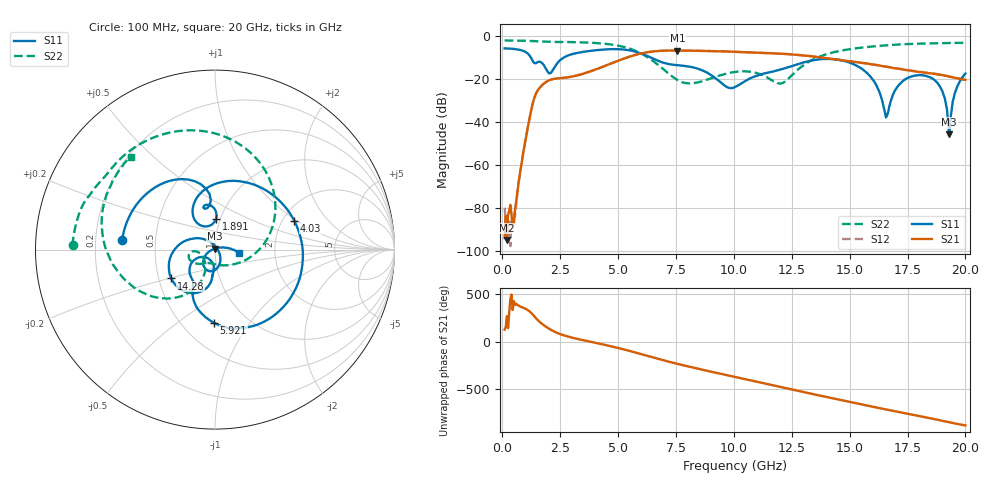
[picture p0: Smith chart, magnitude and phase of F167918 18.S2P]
!  2-Port S-parameters saved by WinCal
! VAR MeasName=S-Parameters (CALIBRATED_DATA) read from VNA (N5242A)
! VAR MeasDate=2016-11-22 10:25:39
! VAR NAME=F167918 18
! VAR FILENAME=F167918 18.S2P
! VAR DATE=2016-11-22 10:25:39
! VAR PHYS_PORTS=1,2
# Hz S DB R 50
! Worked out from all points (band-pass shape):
!   401 points, 100 MHz to 20 GHz, reference 50 ohm
!   highest |S21| = -6.67 dB at 7.562 GHz (marker M1); lowest = -94.7 dB at 199.5 MHz (marker M2)
!   |S21| within 3 dB of the highest: 5.456 GHz to 13.57 GHz (8.112 GHz wide, 85.3 % of centre)
!   lowest |S11| = -45.6 dB at 19.3 GHz (marker M3), VSWR 1.01, Z = 49.7 + j0.456 ohm
!   |S11| at or under -10 dB: 1.238 GHz to 2.646 GHz (1.408 GHz wide, 72.5 % of centre); 6.426 GHz to end of sweep
!   |S22| runs from -22.1 to -2.0 dB; largest |S21 - S12| = 0.0038
!   S11 on the Smith chart (normalised r, x): 100 MHz: 0.32, +0.05; 1.891 GHz: 0.95, +0.34; 4.03 GHz: 2.30, +0.96; 5.921 GHz: 0.71, -0.69; 14.28 GHz: 0.58, -0.20; 20 GHz: 1.31, -0.05
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1e8  -5.68 174.1  -93.87 125.8  -79.76 19.0  -2.00 178.3
1.995e8  -5.72 168.2  -94.73 -92.7  -88.44 4.8  -2.01 176.7
5.4775e8  -6.02 146.9  -80.79 25.2  -84.15 1.8  -2.06 171.0
1.294e9  -11.10 94.9  -32.29 -69.4  -32.26 -69.5  -2.28 158.6
1.891e9  -15.27 87.9  -21.32 155.3  -21.28 155.1  -2.57 149.6
3.43325e9  -7.42 56.6  -17.68 17.8  -17.69 17.6  -2.89 122.4
4.03025e9  -6.56 20.2  -15.51 -13.2  -15.53 -13.2  -3.19 107.9
5.92075e9  -7.80 -90.9  -8.23 -126.7  -8.19 -126.7  -7.64 35.8
6.7665e9  -11.63 -118.6  -6.88 175.7  -6.86 175.7  -13.69 -10.5
7.5625e9  -13.51 -126.2  -6.67 125.6  -6.67 125.6  -20.38 -65.2
1.005e10  -23.70 -111.0  -7.26 -12.7  -7.27 -12.7  -16.64 -153.9
1.204e10  -15.46 -96.5  -8.18 -118.1  -8.14 -118.2  -21.97 -144.2
1.338325e10  -11.30 -117.3  -9.41 168.9  -9.36 169.2  -11.10 -121.0
1.427875e10  -10.70 -146.6  -10.64 122.3  -10.63 122.4  -7.57 -140.3
1.567175e10  -16.37 157.5  -12.58 51.5  -12.64 51.6  -5.16 -166.8
1.656725e10  -37.83 49.9  -14.22 6.5  -14.13 6.9  -4.27 178.8
1.67165e10  -32.64 -24.7  -14.41 -1.1  -14.43 -0.4  -4.17 176.5
1.726375e10  -21.15 -74.3  -15.43 -27.8  -15.34 -26.9  -3.81 168.3
1.825875e10  -18.38 -115.2  -16.98 -75.3  -16.88 -75.2  -3.41 154.1
1.89055e10  -23.44 -146.9  -17.96 -108.1  -17.83 -108.3  -3.27 145.9
1.93035e10  -45.63 118.9  -18.82 -129.2  -18.68 -128.8  -3.19 140.7
2e10  -17.39 -7.9  -20.34 -162.3  -20.22 -162.0  -3.10 132.3
